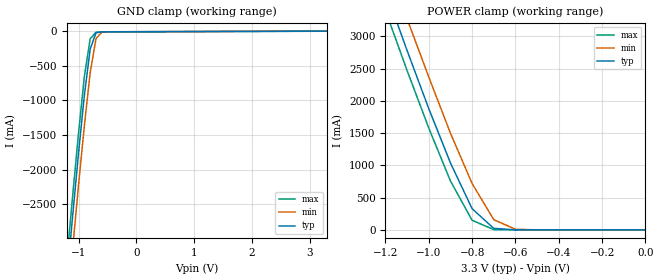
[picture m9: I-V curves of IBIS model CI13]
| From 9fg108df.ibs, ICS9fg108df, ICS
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|   Model CI13
[Model]   CI13
Model_type   Input
Polarity   Non-Inverting
Enable   Active-High
Vinl =   0.80V
Vinh =   2.00V
C_comp   5.50pF   5.00pF   6.00pF
[Temperature Range]   27.00   70.00   0.000
[Voltage Range]   3.30V   3.00V   3.70V
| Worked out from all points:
|   POWER clamp passes 1 mA (typ) near -0.39 V on its own axis
[GND_clamp]
| voltage   I(typ)   I(min)   I(max)
-3.3V     -24.07A    -24.5A     -23.81A
-1.2V     -3.56A     -4.03A     -3.27A
-1.1V     -2.64A     -3.11A     -2.35A
-1V       -1.75A     -2.21A     -1.46A
-900mV    -920mA     -1.36A     -650mA
-800mV    -260mA     -600mA     -110mA
-700mV    -24.92mA   -110mA     -15.24mA
-600mV    -10.96mA   -15.13mA   -11.57mA
-500mV    -9.91mA    -9.4mA     -10.9mA
3.3V      130pA      780uA      -1.03mA
[POWER_clamp]
| voltage   I(typ)   I(min)   I(max)
-3.3V     24.22A     24.67A     23.94A
-1.2V     3.71A      4.2A       3.4A
-1.1V     2.78A      3.27A      2.47A
-1V       1.88A      2.37A      1.58A
-900mV    1.04A      1.5A       760mA
-800mV    330mA      720mA      150mA
-700mV    24.76mA    160mA      5.64mA
-600mV    2.11mA     10.91mA    1.62mA
0V        130pA      310pA      130pA
